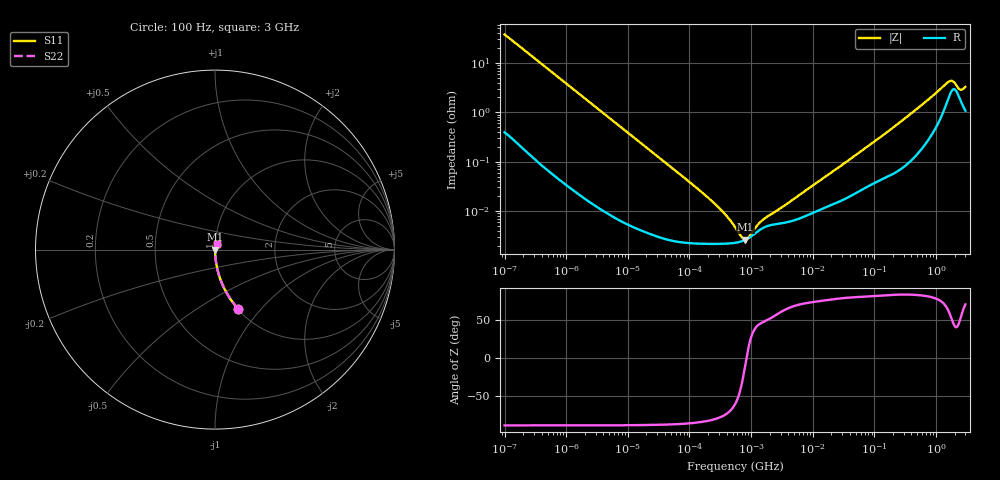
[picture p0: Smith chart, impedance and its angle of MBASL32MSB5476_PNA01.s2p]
! MBASL32MSB5476_PNA01  S-PARAMETER MODEL  ( Standard Model )
! Model Generated by TAIYO YUDEN Corporation (http://www.ty-top.com)
! Version 1.0
! TAIYO YUDEN Control No. 220601
! Copyright(c) 2015 TAIYO YUDEN CO.,LTD. All Rights Reserved.
! Product Description (link to TY-COMPAS)
! https://ds.yuden.co.jp/TYCOMPAS/or/detail?pn=MBASL32MSB5476KPNA01&u=M
! Products Name : Multilayer Ceramic Capacitors
! Characteristics :
!  Capacitance : 47 [uF] , Rated Voltage : 10 [V] , TCC : X5R
!  Case Size : 3.2 x 2.5 / 0.126 x 0.098 [mm/inch] , Thickness : 2.5 / 0.098 [mm/inch]
!  (Conditions: Temperature = 25 [degC] , DC Bias Voltage = 0 [V])
! External Node Assignments :
!  1  o---| |---o  2
! GND o---------o GND
! Frequency Range : 100Hz  -  3GHz  [ 401 STEP ]
# MHZ S RI R 50
! Freq[MHz].  S11 Real  S11 Imag  S21 Real  S21 Imag  S12 Real  S12 Imag  S22 Real  S22 Imag
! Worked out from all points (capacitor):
!   401 points, 100 Hz to 3 GHz, reference 50 ohm
!   read as one part in series: C = 42 uF near 109 Hz
!   lowest |Z| = 2.64 mohm at 806.9 kHz (marker M1)
!   series resonance near 841.5 kHz, so ESL is about 850 pH
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0.0001  0.1278 -0.3287  0.8722 0.3287  0.8722 0.3287  0.1278 -0.3287
0.000175  0.0469 -0.2065  0.9531 0.2065  0.9531 0.2065  0.0469 -0.2065
0.000348  0.0128 -0.108  0.9872 0.108  0.9872 0.108  0.0128 -0.108
0.000724  0.00324 -0.0527  0.9968 0.0527  0.9968 0.0527  0.00324 -0.0527
0.001788  0.000658 -0.0215  0.9993 0.0215  0.9993 0.0215  0.000658 -0.0215
0.031977  3.1e-05 -0.00122  1 0.00122  1 0.00122  3.1e-05 -0.00122
0.144239  2.19e-05 -0.000264  1 0.000264  1 0.000264  2.19e-05 -0.000264
0.326774  2.16e-05 -0.000103  1 0.000103  1 0.000103  2.16e-05 -0.000103
0.371814  2.18e-05 -8.56e-05  1 8.56e-05  1 8.56e-05  2.18e-05 -8.56e-05
0.547723  2.27e-05 -4.18e-05  1 4.18e-05  1 4.18e-05  2.27e-05 -4.18e-05
0.806856  2.61e-05 -3.94e-06  1 3.94e-06  1 3.94e-06  2.61e-05 -3.94e-06
2.579298  5.45e-05 8.44e-05  0.9999 -8.44e-05  0.9999 -8.44e-05  5.45e-05 8.44e-05
3.339322  5.74e-05 0.00011  0.9999 -0.00011  0.9999 -0.00011  5.74e-05 0.00011
9.794414  9.05e-05 0.000309  0.9999 -0.000309  0.9999 -0.000309  9.05e-05 0.000309
175.1444  0.000534 0.00427  0.9995 -0.00427  0.9995 -0.00427  0.000534 0.00427
610.2215  0.00214 0.0145  0.9979 -0.0145  0.9979 -0.0145  0.00214 0.0145
1573.002  0.0194 0.0352  0.9806 -0.0352  0.9806 -0.0352  0.0194 0.0352
1714.41  0.0249 0.0342  0.9751 -0.0342  0.9751 -0.0342  0.0249 0.0342
1868.531  0.029 0.0299  0.971 -0.0299  0.971 -0.0299  0.029 0.0299
2317.205  0.0219 0.0205  0.9781 -0.0205  0.9781 -0.0205  0.0219 0.0205
2525.516  0.0172 0.0223  0.9828 -0.0223  0.9828 -0.0223  0.0172 0.0223
3000  0.0116 0.0304  0.9884 -0.0304  0.9884 -0.0304  0.0116 0.0304
